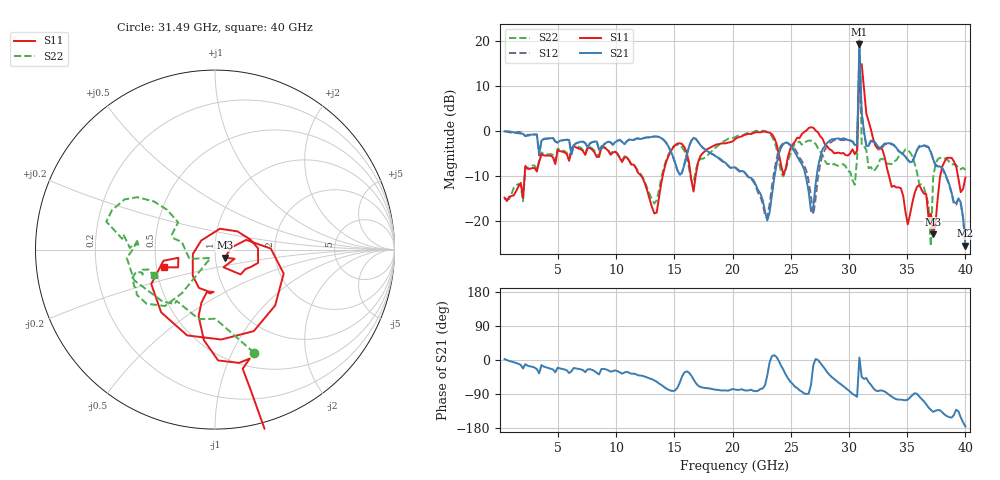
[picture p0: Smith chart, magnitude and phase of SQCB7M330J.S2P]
! Network Analyzer HP8722ES.07.66: Jul 25, 2000 Serial No. US39175408
! 27 Oct 2004  10:27:11
! Frequency  S11  S21  S12  S22
# HZ  S  DB R  50
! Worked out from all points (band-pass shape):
!   201 points, 400 MHz to 40 GHz, reference 50 ohm
!   highest |S21| = 19.28 dB at 30.89 GHz (marker M1); lowest = -25.5 dB at 40 GHz (marker M2)
!   |S21| within 3 dB of the highest: 30.86533 GHz to 30.93068 GHz (65.35 MHz wide, 0.211 % of centre)
!   lowest |S11| = -22.9 dB at 37.23 GHz (marker M3), VSWR 1.15, Z = 55.6 - j5.09 ohm
!   |S11| at or under -10 dB: start of sweep to 2.12 GHz; 12.14 GHz to 13.99 GHz (1.851 GHz wide, 14.2 % of centre); 33.43 GHz to 37.83 GHz (4.4 GHz wide, 12.3 % of centre)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
!   |S22| runs from -25.6 to 20.1 dB; largest |S21 - S12| = 2.9
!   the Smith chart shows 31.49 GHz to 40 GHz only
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4e8  -14.81 -91.7  -0.11 2.5  -0.01 3.6  -15.09 -86.7
7.132e9  -4.46 -121.3  -2.36 -26.6  -2.45 -27.8  -4.26 -109.5
1.3666e10  -14.78 -20.1  -1.33 -61.9  -1.35 -62.3  -13.09 -6.6
1.5844e10  -3.57 -59.7  -7.53 -33.0  -7.41 -32.9  -4.38 -45.5
1.6636e10  -13.45 -30.1  -1.53 -51.2  -1.58 -51.4  -11.43 -8.2
2.02e10  -1.85 -4.2  -8.06 -77.8  -8.17 -77.6  -1.41 6.4
2.2972e10  -0.27 -23.6  -19.86 -41.2  -19.35 -24.5  -0.31 -18.9
2.4358e10  -9.71 -17.5  -2.92 -25.8  -2.70 -29.4  -10.08 -11.2
2.5744e10  -1.59 9.3  -6.59 -80.1  -5.91 -78.4  -2.33 -7.9
2.6932e10  0.71 -8.1  -16.87 -13.3  -18.56 -56.1  -2.61 -73.9
2.7724e10  -1.74 -19.2  -4.06 -15.2  -5.16 -13.4  -5.31 -154.9
3.0694e10  -4.36 8.4  -2.99 -97.2  -2.90 -96.4  -6.06 125.6
3.0892e10  14.02 104.1  19.28 6.7  16.04 2.8  20.06 -106.1
3.109e10  14.81 -6.6  3.92 -44.9  3.91 -47.2  -3.13 -95.1
3.1288e10  9.26 -39.8  -0.13 -50.0  -0.30 -51.6  -3.36 -70.9
3.1684e10  2.12 -66.6  -3.29 -58.7  -3.01 -61.6  -8.28 -89.7
3.3466e10  -10.31 -104.4  -2.73 -92.5  -2.67 -91.7  -7.28 174.9
3.5446e10  -15.86 39.1  -6.81 -92.8  -6.69 -92.3  -5.63 146.1
3.703e10  -18.37 -24.9  -4.75 -131.5  -4.60 -133.7  -25.57 -118.1
3.7228e10  -22.94 -39.7  -6.29 -136.9  -6.13 -139.7  -10.32 -127.2
3.8218e10  -6.80 -42.8  -9.19 -144.1  -9.51 -149.5  -6.11 -155.6
4e10  -10.37 -161.0  -25.47 -175.6  -24.88 170.9  -8.66 -157.6
